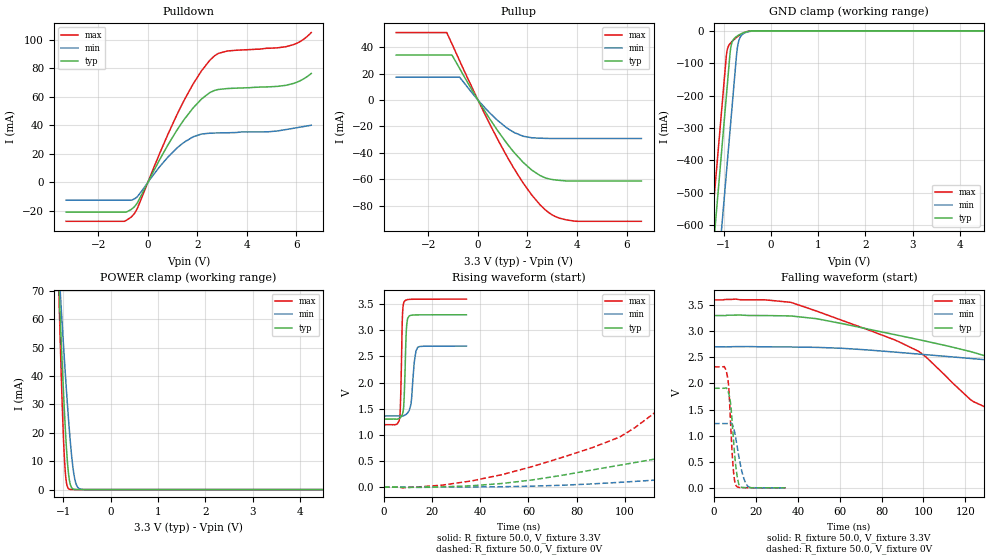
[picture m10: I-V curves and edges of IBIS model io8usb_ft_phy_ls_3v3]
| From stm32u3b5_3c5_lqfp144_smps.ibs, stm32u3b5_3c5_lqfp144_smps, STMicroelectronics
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[Model]   io8usb_ft_phy_ls_3v3
Model_type I/O
Polarity   Non-Inverting
Enable   Active-Low
| CAP_THRESHOLD on pad DPFT is "UDTCAPC" :
| Rising=30.0% of vddiom   Falling=70.0% of vddiom
| C_comp min and max val. don't necessarily correlate with the min and max pvt
| but are the smallest and greatest pad capacitance found.
| var   typ   min   max
C_comp   7.90877pF  7.74428pF  7.91322pF
|C_comp_pullup   5.14486pF  4.79251pF  5.28037pF
|C_comp_pulldown   2.76391pF  2.95177pF  2.63285pF
Vinl = 1.35V
Vinh = 1.8V
Vmeas = 1.65V   | Reference voltage for timing measurements
Cref  = 50.0pF   | Timing specification test load capacitance value
Rref  = 1.0MOhm   | Timing specification test load resistance value
Vref  = 1.815V   | Timing specification test load voltage
[Model Spec]
| TIME_THRESHOLD on pin ZIUSBPV11 is "CMOS" :
| Rising=50.0% of vdd   Falling=50.0% of vdd
Vinl 1.26850V 1.05950V 1.35350V
Vinh 1.77850V 1.50350V 1.88250V
| variable   typ   min   max
[Temperature Range] 25.0 130.0 -40.0
| variable   typ   min   max
[Voltage Range] 3.3V 2.7V 3.6V
| variable   typ   min   max
[POWER Clamp Reference] 3.3V 2.7V 3.6V
| variable   typ   min   max
[GND Clamp Reference] 0V 0V 0V
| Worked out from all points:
|   slope of the pulldown table from 0 to 0.495 V, typ, clamps not added: 30 ohm
|   slope of the pullup table from 0 to 0.495 V, typ, clamps not added: 33.4 ohm
|   GND clamp passes 1 mA (typ) near -0.45 V on its own axis
|   POWER clamp passes 1 mA (typ) near -0.83 V on its own axis
|   rising waveform, R_fixture 50.0, V_fixture 3.3V: 20-80 % time 822ps typ, 1.42ns min, 663ps max; typ from 1.3 V to 3.3 V
|   falling waveform, R_fixture 50.0, V_fixture 3.3V: 20-80 % time 80.2ns typ, 142ns min, 55.8ns max; typ from 3.3 V to 1.3 V
|   rising waveform, R_fixture 50.0, V_fixture 0V: 20-80 % time 89.2ns typ, 170ns min, 59.1ns max; typ from 0 V to 1.91 V
|   falling waveform, R_fixture 50.0, V_fixture 0V: 20-80 % time 2.36ns typ, 3.53ns min, 1.86ns max; typ from 1.91 V to 0.001 V
[POWER Clamp]
-3.3V     1.126A     769.5mA    1.647A
-1.1V     75.38mA    79.63mA    73.18mA
-1.09V    71.2mA     76.8mA     67.14mA
-1.08V    67.05mA    73.98mA    61.2mA
-1.06V    58.89mA    68.38mA    49.67mA
-1.01V    39.47mA    54.71mA    24.03mA
-970mV    25.49mA    44.18mA    9.257mA
-930mV    13.81mA    34.16mA    2.168mA
-870mV    3.251mA    20.56mA    140.6uA
-760mV    67.19uA    3.98mA     740.2nA
-630mV    519.2nA    149uA      2.216nA
6.6V      0A         0A         0A
[GND Clamp]
-3.3V     -4.213A    -4.451A    -4.087A
-1.25V    -727.6mA   -966.1mA   -601.9mA
-950mV    -217.6mA   -456.1mA   -91.89mA
-930mV    -183.6mA   -422.1mA   -65.18mA
-860mV    -66.05mA   -303.1mA   -39.14mA
-840mV    -46.26mA   -269.1mA   -35.85mA
-800mV    -28.83mA   -201.1mA   -30.02mA
-720mV    -16.98mA   -67.05mA   -19.74mA
-670mV    -12.46mA   -27.4mA    -14.18mA
-590mV    -6.767mA   -9.636mA   -7.036mA
-220mV    -696.1nA   -13.77uA   -55.48nA
6.6V      4.659nA    635.5nA    2.057nA
| variable   typ   min   max
[Pullup Reference] 3.3V 2.7V 3.6V
| variable   typ   min   max
[Pulldown Reference] 0V 0V 0V
[Pullup]
-3.3V     34.01mA    17.25mA    51.02mA
-1.26V    34.01mA    17.25mA    51.02mA
-1.05V    34.01mA    17.25mA    42.54mA
-740mV    23.86mA    17.25mA    29.69mA
460mV     -13.82mA   -9.49mA    -17.59mA
1.14V     -32.15mA   -20.75mA   -41.66mA
1.83V     -47.29mA   -27.48mA   -62.97mA
2.17V     -53.01mA   -28.6mA    -71.87mA
2.82V     -59.5mA    -29.12mA   -84.67mA
3.3V      -60.88mA   -29.17mA   -89.51mA
3.95V     -61.36mA   -29.17mA   -91.8mA
6.6V      -61.36mA   -29.17mA   -91.85mA
[Pulldown]
-3.3V     -20.77mA   -12.37mA   -27.2mA
-950mV    -20.77mA   -12.37mA   -27.2mA
-570mV    -17.45mA   -11.78mA   -22.39mA
-410mV    -13.9mA    -9.674mA   -17.62mA
800mV     25.93mA    17.54mA    33.25mA
1.3V      39.9mA     25.91mA    51.82mA
2.17V     58.5mA     33.95mA    78.26mA
2.7V      64.53mA    34.65mA    88.8mA
3.19V     65.78mA    34.82mA    92.02mA
5.58V     68.09mA    37.06mA    95.13mA
6.13V     71.09mA    38.7mA     98.53mA
6.6V      76.36mA    40.11mA    105mA
[Ramp]
dV/dt_r 1.14478V/89.18862ns 739.34088mV/169.54784ns 1.39063V/58.55452ns
dV/dt_f 1.19875V/80.14875ns 803.25981mV/141.24419ns 1.44295V/55.7438ns
R_load = 50.0
| Removed startup time: 0s 0s 0s  .
| Removed end time: 34.25ns.
[Rising Waveform]
R_fixture   = 50.0
V_fixture   = 3.3V
V_fixture_min = 2.7V
V_fixture_max = 3.6V
0s        1.302V     1.361V     1.195V
6.6ns     1.322V     1.361V     1.347V
6.95ns    1.336V     1.36V      1.739V
7.7ns     1.401V     1.361V     3.293V
8.45ns    1.784V     1.372V     3.552V
9.35ns    3.037V     1.398V     3.583V
10.5ns    3.277V     1.468V     3.593V
12.6ns    3.295V     2.393V     3.596V
14ns      3.296V     2.675V     3.596V
34.25ns   3.298V     2.699V     3.598V
| Removed startup time: 0s 0s 0s  .
| Removed end time: 599.25ns.
[Falling Waveform]
R_fixture   = 50.0
V_fixture   = 3.3V
V_fixture_min = 2.7V
V_fixture_max = 3.6V
0s        3.3V       2.7V       3.6V
36.7ns    3.292V     2.698V     3.553V
73.4ns    3.043V     2.642V     3.03V
97.85ns   2.838V     2.562V     2.612V
123.9ns   2.595V     2.474V     1.652V
159ns     1.959V     2.347V     1.254V
183.4ns   1.518V     2.249V     1.201V
207.9ns   1.381V     2.132V     1.196V
330.3ns   1.302V     1.431V     1.195V
599.3ns   1.302V     1.361V     1.195V
| Removed startup time: 0s 0s 0s  .
| Removed end time: 599.25ns.
[Rising Waveform]
R_fixture   = 50.0
V_fixture   = 0V
V_fixture_min = 0V
V_fixture_max = 0V
0s        35.13nV    302.2nV    81.71nV
24.45ns   5.028mV    -71.88uV   39.11mV
61.15ns   134.5mV    17.89mV    387.3mV
97.85ns   419.3mV    91.33mV    957.3mV
127.7ns   670.8mV    178.5mV    1.908V
169.8ns   1.307V     303.8mV    2.264V
195.7ns   1.682V     387.6mV    2.303V
244.6ns   1.87V      573.6mV    2.316V
366.9ns   1.907V     1.152V     2.318V
599.3ns   1.908V     1.232V     2.318V
| Removed startup time: 0s 0s 0s  .
| Removed end time: 34.2ns.
[Falling Waveform]
R_fixture   = 50.0
V_fixture   = 0V
V_fixture_min = 0V
V_fixture_max = 0V
0s        1.908V     1.232V     2.318V
4.9ns     1.909V     1.232V     2.323V
6.3ns     1.889V     1.233V     2.152V
7.05ns    1.798V     1.237V     1.899V
7.85ns    1.627V     1.241V     1.269V
9.1ns     1.009V     1.175V     401.7mV
10.5ns    373.8mV    919.1mV    41.91mV
11.9ns    62.88mV    586.5mV    9.144mV
16.1ns    3.082mV    31.76mV    3.304mV
34.2ns    1.415mV    802.5uV    1.915mV
